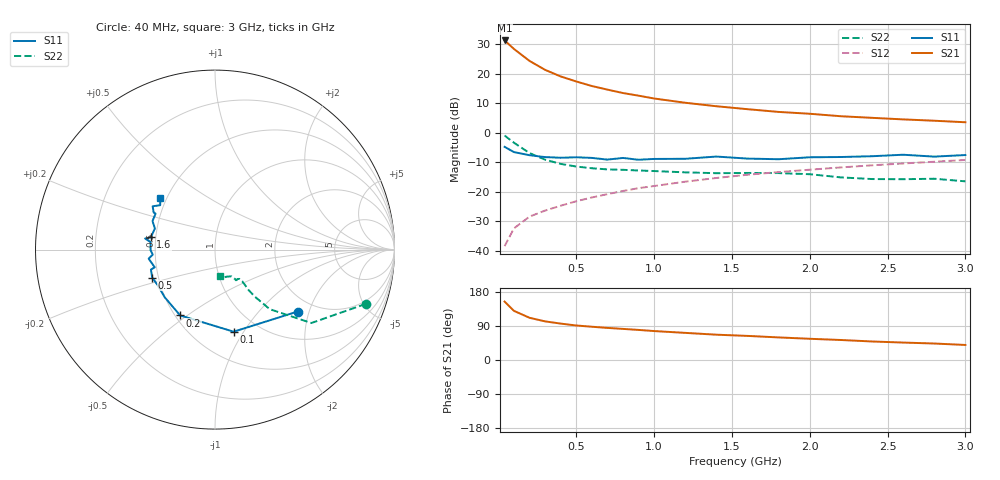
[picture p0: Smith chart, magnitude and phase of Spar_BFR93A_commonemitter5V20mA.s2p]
! Filename:  BFR93AC.S2P  Version:  2.0
! NXP part #: BFR93A  Date: May 1990
! Bias condition: Vce=5V, Ic=20mA
#  MHz  S  MA  R  50
! Freq  S11  S21  S12  S22  !GUM [dB]
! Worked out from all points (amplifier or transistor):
!   21 points, 40 MHz to 3 GHz, reference 50 ohm
!   highest |S21| = 31.2 dB at 40 MHz (marker M1)
!   |S21| within 3 dB of that: start of sweep to 103.1 MHz
!   unconditionally stable (mu >= 1): 671.5 MHz to 793.2 MHz; 803.2 MHz to 2.512 GHz; 2.704 GHz to 2.908 GHz
!   at 300 MHz: K = 0.82, MSG = 23.8 dB, |S12| = -26.4 dB
!   at 1 GHz: K = 1.03, MAG = 13.7 dB, |S12| = -18.1 dB
!   at 3 GHz: K = 0.99, MSG = 6.4 dB, |S12| = -9.2 dB
!   S11 on the Smith chart (normalised r, x): 40 MHz: 1.63, -1.68; 100 MHz: 0.77, -0.90; 200 MHz: 0.53, -0.47; 500 MHz: 0.46, -0.17; 1.6 GHz: 0.47, +0.07; 3 GHz: 0.46, +0.32
40  0.575 -36.9  36.29 154.1  0.012 74.7  0.893 -19.8
100  0.469 -77.2  26.07 129.7  0.024 61.3  0.675 -37.3
200  0.415 -117.9  16.36 111.4  0.038 61.4  0.451 -47.4
300  0.386 -136.5  11.55 101.9  0.048 63.3  0.349 -49.6
400  0.376 -147.9  8.937 96.1  0.058 65.4  0.296 -50.3
500  0.383 -156.0  7.343 91.1  0.069 67.4  0.267 -49.9
600  0.374 -162.7  6.156 87.8  0.08 68.3  0.25 -49.6
700  0.35 -163.6  5.347 84.7  0.091 70.0  0.239 -49.6
800  0.373 -172.2  4.681 82.1  0.103 69.8  0.235 -49.2
900  0.348 -175.4  4.224 79.4  0.115 70.2  0.229 -49.4
1000  0.359 -179.5  3.783 76.4  0.125 70.6  0.224 -49.1
1200  0.361 173.4  3.205 71.6  0.148 70.4  0.213 -50.0
1400  0.394 171.0  2.798 66.8  0.171 69.2  0.206 -52.8
1600  0.364 169.2  2.495 63.6  0.194 69.1  0.208 -54.2
1800  0.355 160.6  2.242 59.6  0.215 67.6  0.207 -55.6
2000  0.383 155.4  2.087 56.0  0.236 66.3  0.198 -55.8
2200  0.387 148.8  1.895 52.8  0.258 65.8  0.175 -58.4
2400  0.399 148.9  1.781 48.9  0.28 64.4  0.164 -66.7
2600  0.423 145.2  1.676 46.0  0.301 62.7  0.163 -73.5
2800  0.393 141.0  1.591 43.5  0.322 61.5  0.166 -77.0
3000  0.418 136.6  1.499 39.7  0.345 59.8  0.15 -79.5
